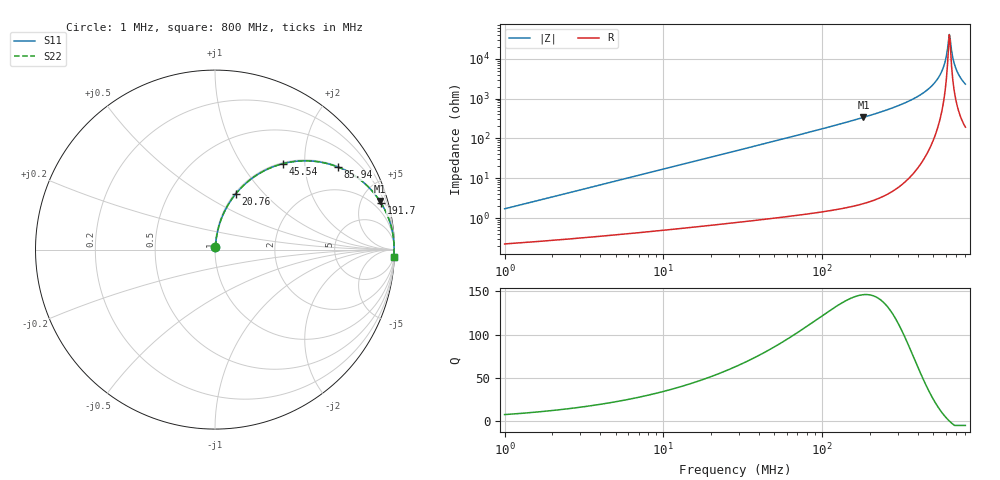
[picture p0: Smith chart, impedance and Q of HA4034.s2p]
# MHz S MA R 50
!Freq  MagS11  AngS11  MagS21  AngS21  MagS12  AngS12  MagS22  AngS22
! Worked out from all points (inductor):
!   801 points, 1 MHz to 800 MHz, reference 50 ohm
!   read as one part in series: L = 270 nH near 1.034 MHz
!   highest Q = 146 at 182.3 MHz (marker M1), where L = 294 nH
!   self-resonance near 633.1 MHz
!   S11 on the Smith chart (normalised r, x): 1 MHz: 1.00, +0.03; 20.76 MHz: 1.01, +0.71; 45.54 MHz: 1.02, +1.55; 85.94 MHz: 1.03, +2.97; 191.7 MHz: 1.05, +7.16; 800 MHz: 5, -46
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1  0.01707 81.5  0.9976 -1.0  0.9976 -1.0  0.01707 81.5
3.063851  0.05184 83.5  0.9955 -3.0  0.9955 -3.0  0.05184 83.5
9.30907  0.1554 79.3  0.9831 -8.9  0.9831 -8.9  0.1554 79.3
20.76238  0.3306 69.6  0.9375 -19.3  0.9375 -19.3  0.3306 69.6
28.28427  0.4307 63.6  0.8957 -25.5  0.8957 -25.5  0.4307 63.6
45.5397  0.6098 51.7  0.7851 -37.6  0.7851 -37.6  0.6098 51.7
85.9377  0.8261 33.8  0.5562 -55.7  0.5562 -55.7  0.8261 33.8
86.65878  0.8284 33.6  0.5529 -55.9  0.5529 -55.9  0.8284 33.6
182.2978  0.9569 16.5  0.2839 -73.1  0.2839 -73.1  0.9569 16.5
191.6702  0.9614 15.6  0.2687 -74.0  0.2687 -74.0  0.9614 15.6
263.3003  0.9819 10.5  0.182 -79.1  0.182 -79.1  0.9819 10.5
389.949  0.9942 5.4  0.09355 -83.8  0.09355 -83.8  0.9942 5.4
501.0415  0.9973 2.5  0.04423 -85.2  0.04423 -85.2  0.9973 2.5
572.711  0.9977 1.1  0.01919 -82.7  0.01919 -82.7  0.9977 1.1
597.145  0.9977 0.6  0.01152 -78.3  0.01152 -78.3  0.9977 0.6
622.6215  0.9976 0.2  0.004267 -56.4  0.004267 -56.4  0.9976 0.2
633.1139  0.9976 0.0  0.002458 -10.9  0.002458 -10.9  0.9976 0.0
649.1849  0.9975 -0.2  0.004874 58.7  0.004874 58.7  0.9975 -0.2
676.8816  0.9972 -0.7  0.01222 76.6  0.01222 76.6  0.9972 -0.7
705.76  0.9969 -1.1  0.01988 80.5  0.01988 80.5  0.9969 -1.1
748.2713  0.9963 -1.8  0.03074 82.3  0.03074 82.3  0.9963 -1.8
800  0.9955 -2.5  0.04329 82.8  0.04329 82.8  0.9955 -2.5
